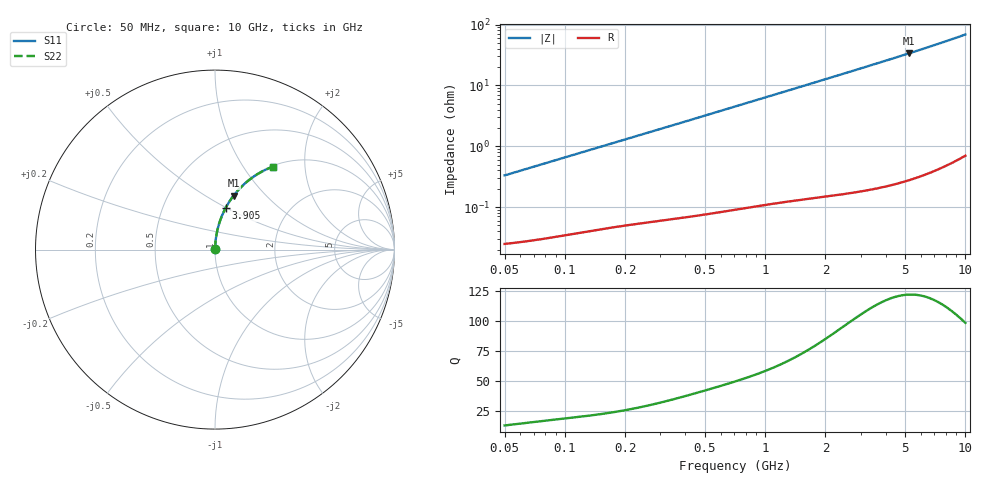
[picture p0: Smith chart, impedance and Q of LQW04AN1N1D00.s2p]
!Murata Part Number: LQW04AN1N1D00
!These Parameters are Measured in Series Mode Connection
!  o--[Z]--o
!Port1  Port2
!  o-------o
!Freq. Start=50[MHz] Stop=10[GHz], 401[Steps]
# Hz S RI R 50
!Freq.(Hz)	S 11(Real)	S 11(Imag)	S 21(Real)	S 21(Imag)	S 12(Real)	S 12(Imag)	S 22(Real)	S 22(Imag)
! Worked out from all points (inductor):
!   401 points, 50 MHz to 10 GHz, reference 50 ohm
!   read as one part in series: L = 1.05 nH near 51.34 MHz
!   highest Q = 122 at 5.225 GHz (marker M1), where L = 1.02 nH
!   S11 on the Smith chart (normalised r, x): 50 MHz: 1.00, +0.01; 3.905 GHz: 1.00, +0.50; 10 GHz: 1.01, +1.37
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5e7  0.000259 0.0033  0.9997 -0.0033  0.9997 -0.0033  0.000259 0.0033
5.134228e7  0.000262 0.00339  0.9997 -0.00339  0.9997 -0.00339  0.000262 0.00339
1.214486e8  0.000445 0.00791  0.9996 -0.00791  0.9996 -0.00791  0.000445 0.00791
2.949953e8  0.000948 0.0189  0.9991 -0.0189  0.9991 -0.0189  0.000948 0.0189
4.689809e8  0.00162 0.0298  0.9984 -0.0298  0.9984 -0.0298  0.00162 0.0298
7.071068e8  0.00291 0.0447  0.9971 -0.0447  0.9971 -0.0447  0.00291 0.0447
1.139142e9  0.0063 0.0715  0.9937 -0.0715  0.9937 -0.0715  0.0063 0.0715
1.408053e9  0.0091 0.088  0.9909 -0.088  0.9909 -0.088  0.0091 0.088
1.717543e9  0.013 0.1069  0.987 -0.1069  0.987 -0.1069  0.013 0.1069
2.122994e9  0.0191 0.1313  0.9809 -0.1313  0.9809 -0.1313  0.0191 0.1313
2.624158e9  0.0284 0.161  0.9716 -0.161  0.9716 -0.161  0.0284 0.161
3.243629e9  0.0422 0.1966  0.9578 -0.1966  0.9578 -0.1966  0.0422 0.1966
3.904516e9  0.0599 0.2331  0.9401 -0.2331  0.9401 -0.2331  0.0599 0.2331
4.171863e9  0.0679 0.2474  0.9321 -0.2474  0.9321 -0.2474  0.0679 0.2474
4.700058e9  0.0849 0.2747  0.9151 -0.2747  0.9151 -0.2747  0.0849 0.2747
5.225452e9  0.1034 0.3005  0.8966 -0.3005  0.8966 -0.3005  0.1034 0.3005
6.207365e9  0.1419 0.3448  0.8581 -0.3448  0.8581 -0.3448  0.1419 0.3448
7.276762e9  0.1886 0.3869  0.8114 -0.3869  0.8114 -0.3869  0.1886 0.3869
8.307378e9  0.2374 0.4209  0.7626 -0.4209  0.7626 -0.4209  0.2374 0.4209
8.994549e9  0.2714 0.4399  0.7286 -0.4399  0.7286 -0.4399  0.2714 0.4399
9.738562e9  0.3092 0.4572  0.6908 -0.4572  0.6908 -0.4572  0.3092 0.4572
1e10  0.3226 0.4624  0.6774 -0.4624  0.6774 -0.4624  0.3226 0.4624
